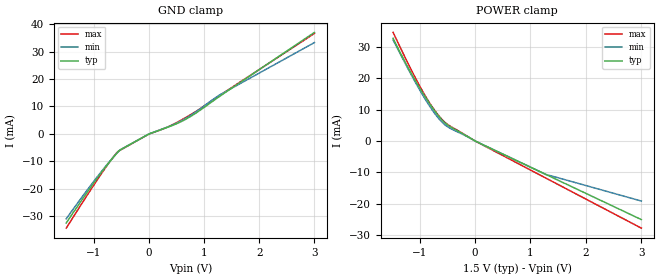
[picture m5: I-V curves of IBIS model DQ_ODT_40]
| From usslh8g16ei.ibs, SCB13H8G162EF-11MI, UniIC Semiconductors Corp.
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|   Model DQ_ODT_40
[Model] DQ_ODT_40
Model_type Input
Polarity   Non-Inverting
Enable   Active-High
Vinl =  0.615V
Vinh =  0.885V
C_comp   0.999pF   0.958pF   1.014pF
C_comp_power_clamp   0.660pF   0.619pF   0.673pF
C_comp_gnd_clamp   0.338pF   0.338pF   0.341pF
[Model Spec]
Vinh   0.885V   0.776V   0.922V
Vinl   0.615V   0.506V   0.652V
[Temperature Range]   45.000   95.000   -40.000
[Voltage Range]   1.500V   1.283V   1.575V
[C Comp Corner]
C_comp_power_clamp   0.673pF   0.619pF   0.660pF
C_comp_gnd_clamp   0.341pF   0.338pF   0.338pF
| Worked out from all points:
|   GND clamp passes 1 mA (typ) near -0.09 V on its own axis
|   POWER clamp passes 1 mA (typ) near -0.09 V on its own axis
[GND_clamp]
|Voltage   I(typ)   I(min)   I(max)
-1.5V     -32.4mA    -30.88mA   -34.27mA
-1.159V   -22.35mA   -21.46mA   -23.5mA
-880mV    -14.5mA    -14.14mA   -14.96mA
-725mV    -10.42mA   -10.29mA   -10.51mA
-570mV    -6.705mA   -6.747mA   -6.506mA
-508mV    -5.648mA   -5.632mA   -5.766mA
-12mV     -133.4uA   -133uA     -136.2uA
391mV     2.837mA    2.963mA    3.018mA
577mV     4.432mA    4.688mA    4.967mA
763mV     6.473mA    6.849mA    7.129mA
1.29V     13.81mA    14.3mA     14.13mA
3V        36.96mA    33.26mA    36.58mA
[POWER_clamp]
|Voltage   I(typ)   I(min)   I(max)
-1.476V   32.7mA     32.19mA    34.58mA
-1.166V   22.05mA    21.65mA    23.24mA
-1.011V   17.26mA    16.7mA     17.96mA
-887mV    13.73mA    13.01mA    14.08mA
-763mV    10.46mA    9.68mA     10.65mA
-670mV    8.241mA    7.486mA    8.426mA
-577mV    6.348mA    5.686mA    6.528mA
-484mV    4.951mA    4.409mA    5.128mA
12mV      -100.2uA   -99.99uA   -111.1uA
1.283V    -10.71mA   -10.69mA   -11.88mA
3V        -25.05mA   -19.14mA   -27.77mA
